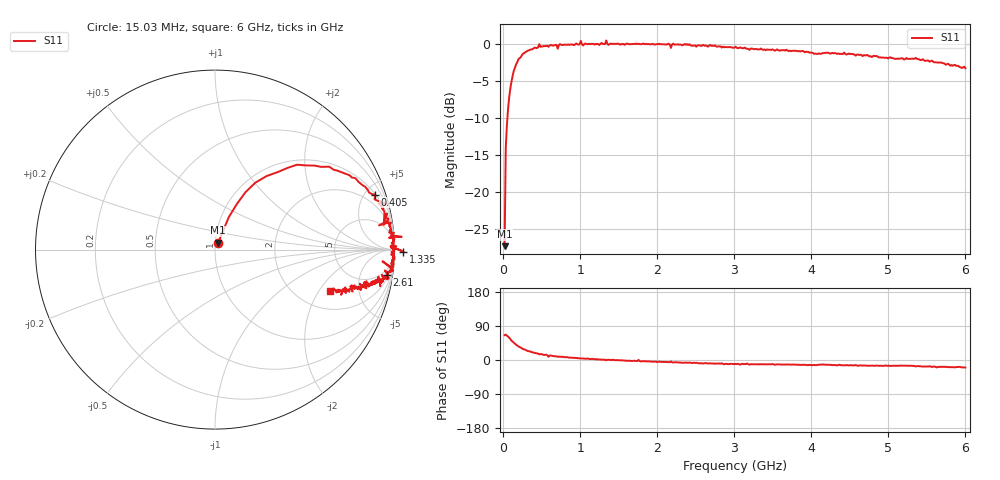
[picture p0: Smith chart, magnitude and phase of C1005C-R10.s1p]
!	Network	Analyzer	HP8753E.07.74:	Oct	30	2002	Serial	No.	JP38451487
!	Hewlett-Packard
!	28	Aug	2009	9:29:53
!	Frequency	S11
#	HZ	S	RI	R	50
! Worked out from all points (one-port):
!   400 points, 15.03 MHz to 6 GHz, reference 50 ohm
!   lowest |S11| = -27.3 dB at 15.03 MHz (marker M1), VSWR 1.09, Z = 51.7 + j4.06 ohm
!   |S11| at or under -10 dB: start of sweep to 51.55 MHz
!   S11 on the Smith chart (normalised r, x): 15.03 MHz: 1.03, +0.08; 405 MHz: 1.10, +5.78; 1.335 GHz: -39, -9; 2.61 GHz: 3, -13; 6 GHz: 2.94, -2.55
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1.502992e7  0.0178 0.0392
3.002985e7  0.077 0.181
6.00297e7  0.171 0.321
9.002955e7  0.288 0.41
1.95029e8  0.636 0.462
4.05028e8  0.889 0.306
4.650277e8  0.959 0.253
5.550272e8  0.934 0.234
5.850271e8  0.941 0.138
6.150269e8  0.959 0.2
7.650262e8  0.965 0.149
9.750251e8  0.98 0.0794
1.005025e9  1.04 0.0712
1.035025e9  0.969 0.0664
1.245024e9  0.978 0.0189
1.335023e9  1.05 -0.0113
1.365023e9  0.98 0.0123
1.515022e9  0.983 -0.0137
1.755021e9  0.997 0.00409
2.145019e9  0.993 -0.0987
2.175019e9  0.933 -0.065
2.265019e9  0.983 -0.109
2.610017e9  0.957 -0.143
3.015015e9  0.937 -0.177
3.765011e9  0.875 -0.183
4.515007e9  0.83 -0.202
5.265004e9  0.762 -0.208
6e9  0.642 -0.231
